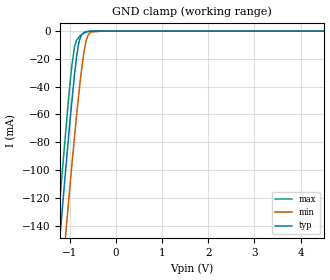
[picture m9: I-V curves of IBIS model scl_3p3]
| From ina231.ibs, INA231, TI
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|   scl_3p3 Model
[Model]   scl_3p3
Model_type   Input
Vinl = 0.4
Vinh = 1.4
|   typ   min   max
|   (nom PVT)   (fast PVT)   (slow PVT)
|C_comp from frequency sweep method (F=100KHz)
|Average
|C_comp   2.156e-12   1.697e-12   2.673e-12
|C_comp from LC tank measurement(L=1nH)
|Average
|Resonant Frequency(Hz)   5.290e+09   5.330e+09   5.240e+09
C_comp   9.061e-13   8.925e-13   9.234e-13
| Where nom  PVT is Nominal Process, 3.3V, 27C
|   Fast PVT is Strong Process,  3.6V, -40C
|   Slow PVT is Weak Process,   3V, 125C
[Voltage Range]   3.3   3   3.6
|Ambient Temperature   25   150   -65
|Junction Temperature
[Temperature Range]   27   125   -40
[Power Clamp Reference]   3.3   3   3.6
[GND Clamp Reference]   0   0   0
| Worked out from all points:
|   GND clamp passes 1 mA (typ) near -0.68 V on its own axis
[GND Clamp]
|   Voltage   I(typ)   I(min)   I(max)
-3.3V     -1.022A    -1.045A    -1.013A
-1.287V   -178.8mA   -223.8mA   -153mA
-1.17V    -132.3mA   -178.2mA   -105.1mA
-1.115V   -110.7mA   -157.5mA   -83.81mA
-1.037V   -81.03mA   -127.7mA   -53.37mA
-954mV    -51.13mA   -96.99mA   -25.24mA
-896.4mV  -31.58mA   -76.47mA   -11.51mA
-785.4mV  -6.119mA   -39.93mA   -3.743mA
-673.2mV  -803.4uA   -11.8mA    -1.034mA
-579mV    -178.8uA   -1.9mA     -338.6uA
-285mV    -18.95uA   -1.068uA   -1.545uA
6.6V      0A         0A         0A
[POWER Clamp]
|   Voltage   I(typ)   I(min)   I(max)
-3.3V     0A         0A         0A
-3.298V   0A         0A         0A
6.6V      0A         0A         0A
